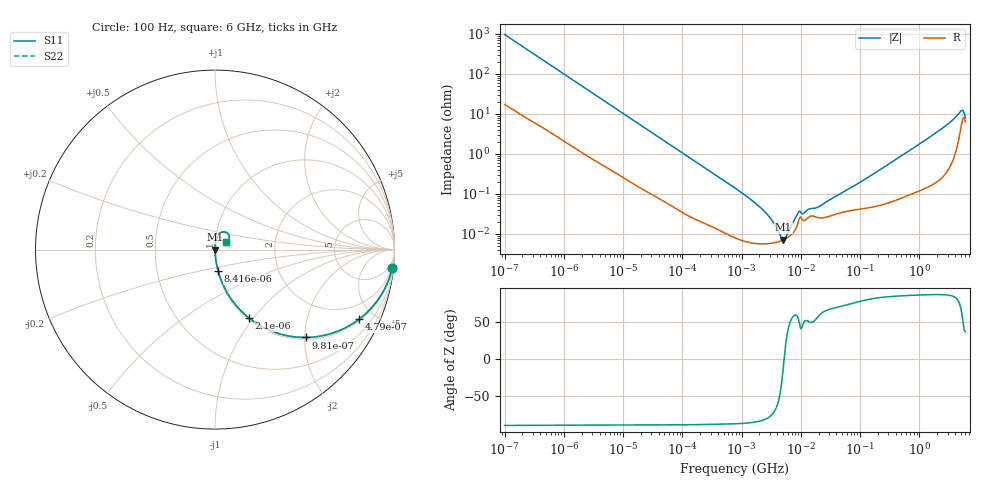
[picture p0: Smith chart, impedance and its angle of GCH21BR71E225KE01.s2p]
!Murata Part Number: GCH21BR71E225KE01
!These Parameters are Measured in Series Mode Connection
!Data Generated on Jun 19, 2026
!  o--ll--o
!Port1  Port2
!  o------o
!Operation Temp=25[degC], DC Bias Voltage=0[V]
!Freq. Start=100[Hz] Stop=6[GHz] 401[Steps]
# Hz S RI R 50
!Freq.(Hz) S11(Real) S11(Imag) S21(Real) S21(Imag) S12(Real) S12(Imag) S22(Real) S22(Imag)
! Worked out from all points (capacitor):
!   401 points, 100 Hz to 6 GHz, reference 50 ohm
!   read as one part in series: C = 1.65 uF near 109 Hz
!   lowest |Z| = 7.27 mohm at 5.079 MHz (marker M1)
!   series resonance near 5.224 MHz, so ESL is about 560 pH
!   S11 on the Smith chart (normalised r, x): 100 Hz: 1, -19; 479 Hz: 1.08, -4.10; 981 Hz: 1.04, -2.02; 2.1 kHz: 1.02, -0.95; 8.416 kHz: 1.01, -0.24; 6 GHz: 1.13, +0.09
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100  0.9875 -0.1024  0.0125 0.1024  0.0125 0.1024  0.9875 -0.1024
245  0.9366 -0.2345  0.0634 0.2345  0.0634 0.2345  0.9366 -0.2345
479  0.8026 -0.3879  0.1974 0.3879  0.1974 0.3879  0.8026 -0.3879
981  0.5051 -0.4895  0.4949 0.4895  0.4949 0.4895  0.5051 -0.4895
2008  0.2041 -0.3923  0.7959 0.3923  0.7959 0.3923  0.2041 -0.3923
2100  0.1905 -0.3819  0.8095 0.3819  0.8095 0.3819  0.1905 -0.3819
3759  0.0721 -0.2476  0.9279 0.2476  0.9279 0.2476  0.0721 -0.2476
8416  0.0174 -0.1189  0.9826 0.1189  0.9826 0.1189  0.0174 -0.1189
40335  0.00145 -0.0259  0.9986 0.0259  0.9986 0.0259  0.00145 -0.0259
774597  8.19e-05 -0.00141  0.9999 0.00141  0.9999 0.00141  8.19e-05 -0.00141
2169299  5.67e-05 -0.000429  0.9999 0.000429  0.9999 0.000429  5.67e-05 -0.000429
3103719  5.84e-05 -0.000236  0.9999 0.000236  0.9999 0.000236  5.84e-05 -0.000236
4246196  6.47e-05 -9.1e-05  0.9999 9.1e-05  0.9999 9.1e-05  6.47e-05 -9.1e-05
5079039  7.16e-05 -1.23e-05  0.9999 1.23e-05  0.9999 1.23e-05  7.16e-05 -1.23e-05
6075234  8.29e-05 6.79e-05  0.9999 -6.79e-05  0.9999 -6.79e-05  8.29e-05 6.79e-05
9090158  0.000202 0.000283  0.9998 -0.000283  0.9998 -0.000283  0.000202 0.000283
1.555665e7  0.000283 0.00033  0.9997 -0.00033  0.9997 -0.00033  0.000283 0.00033
2.128304e7  0.000251 0.000438  0.9997 -0.000438  0.9997 -0.000438  0.000251 0.000438
3.124326e8  0.00064 0.00568  0.9994 -0.00568  0.9994 -0.00568  0.00064 0.00568
2.240541e9  0.00385 0.0395  0.9962 -0.0395  0.9962 -0.0395  0.00385 0.0395
5.016141e9  0.0515 0.0992  0.9485 -0.0992  0.9485 -0.0992  0.0515 0.0992
6e9  0.0613 0.0419  0.9387 -0.0419  0.9387 -0.0419  0.0613 0.0419
